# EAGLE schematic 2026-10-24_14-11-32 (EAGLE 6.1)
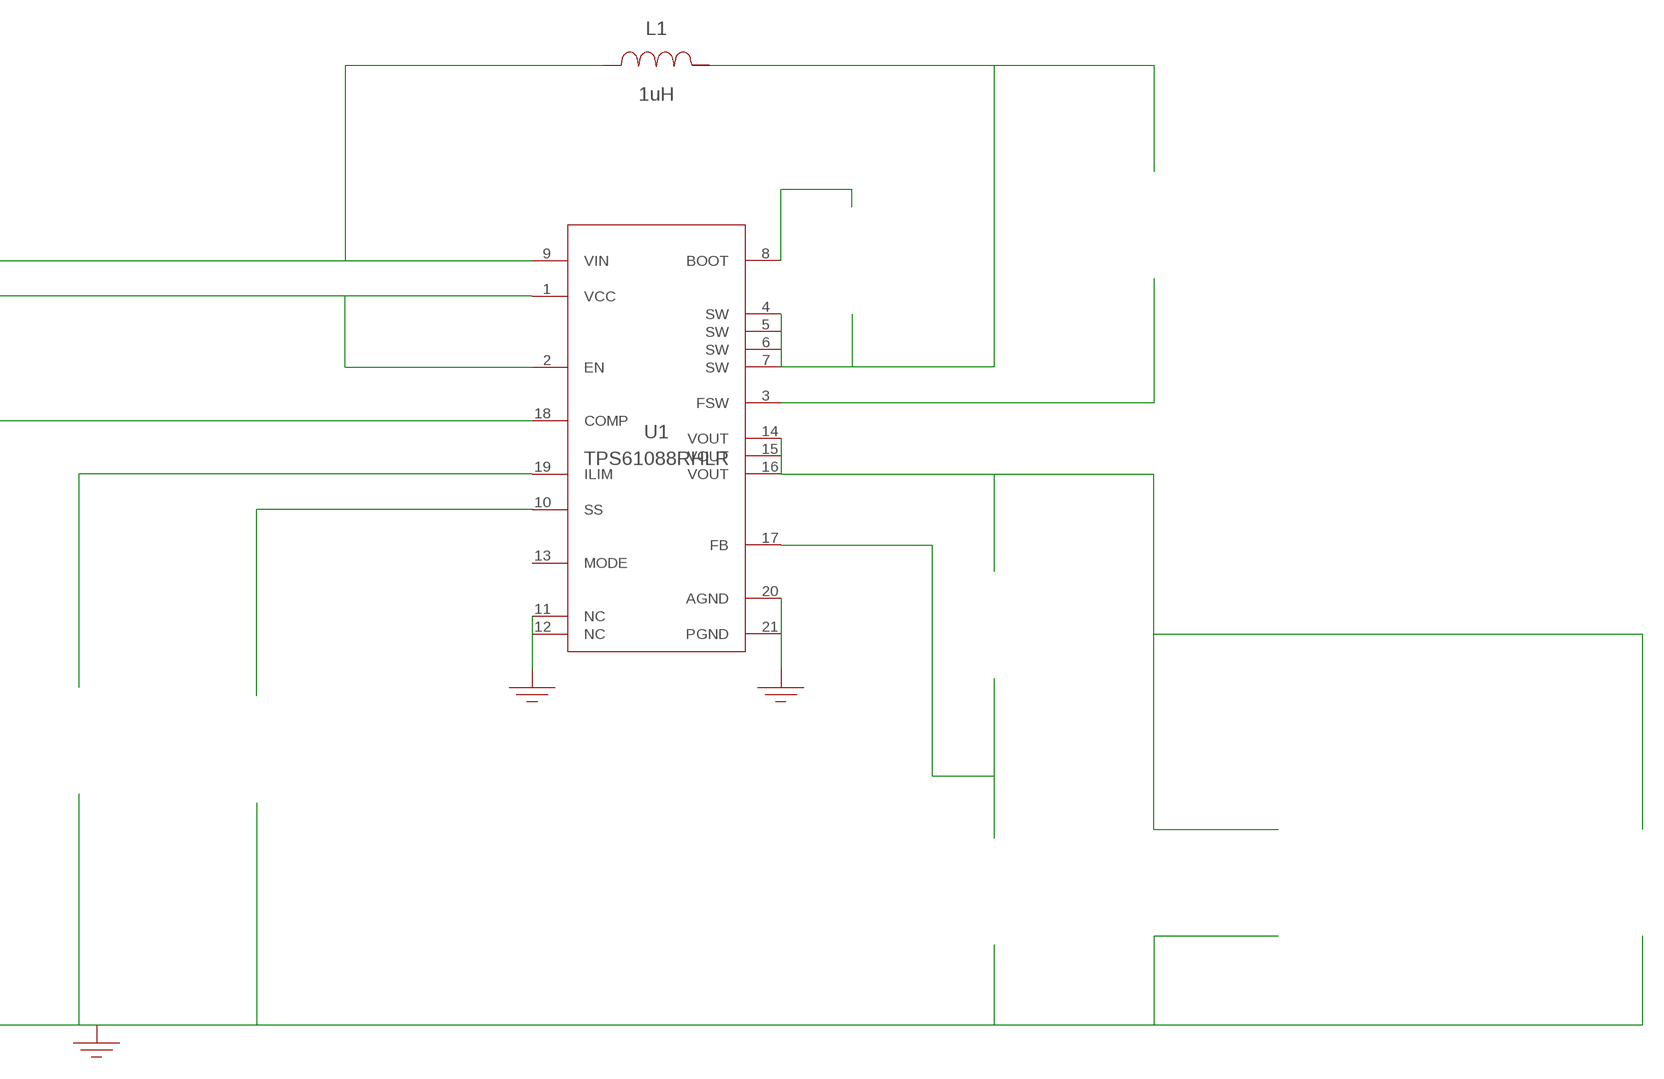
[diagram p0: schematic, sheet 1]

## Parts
CBST  100nF  08053C104KAT2A08053C104KAT2A  [0805]  (not placed on a sheet)
CCOMP  750pF  GRM1555C1E751JA01DGRM1555C1E751JA01D  [0402]  (not placed on a sheet)
CCOMP2  39pF  GRM1555C1E390JA01DGRM1555C1E390JA01D  [0402]  (not placed on a sheet)
CIN  10uF  MSASE21GAB5106KTNA01MSASE21GAB5106KTNA01  [0805]  (not placed on a sheet)
CIN2  100nF  GRM155R71A104KA01DGRM155R71A104KA01D  [0402]  (not placed on a sheet)
CIN_2  10uF  MSASE21GAB5106KTNA01MSASE21GAB5106KTNA01  [0805]  (not placed on a sheet)
CIN_3  10uF  MSASE21GAB5106KTNA01MSASE21GAB5106KTNA01  [0805]  (not placed on a sheet)
COUT  47uF  GRM32ER61C476KE15LGRM32ER61C476KE15L  [1210_280]  (not placed on a sheet)
COUT_2  47uF  GRM32ER61C476KE15LGRM32ER61C476KE15L  [1210_280]  (not placed on a sheet)
CSS  8.2nF  GRM155R71C822KA01DGRM155R71C822KA01D  [0402]  (not placed on a sheet)
CVCC  1uF  EMK107B7105KA-TEMK107B7105KA-T  [0603]  (not placed on a sheet)
CVCC_2  1uF  EMK107B7105KA-TEMK107B7105KA-T  [0603]  (not placed on a sheet)
GND1  WB_GND  WB_GNDWB_GND  [WB_GND]
GND2  WB_GND  WB_GNDWB_GND  [WB_GND]
GND3  WB_GND  WB_GNDWB_GND  [WB_GND]
IOUT  WB_CURRENT_LOAD  WB_CURRENT_LOADWB_CURRENT_LOAD  [WB_CURRENT_LOAD]  (not placed on a sheet)
L1  1uH  VLP8040T-1R0NVLP8040T-1R0N  [VLP8040]
RCOMP  26.7k  CRCW040226K7FKEDCRCW040226K7FKED  [0402]  (not placed on a sheet)
RFBB  69.8k  CRCW040269K8FKEDCRCW040269K8FKED  [0402]  (not placed on a sheet)
RFBT  220k  RC0603FR-07220KLRC0603FR-07220KL  [0603]  (not placed on a sheet)
RLIM  154k  CRCW0402154KFKEDCRCW0402154KFKED  [0402]  (not placed on a sheet)
RT  267k  CRCW0402267KFKEDCRCW0402267KFKED  [0402]  (not placed on a sheet)
U1  TPS61088RHLR  TPS61088RHLRTPS61088RHLR  [RHL0020A]
VIN  WB_BATTERY  WB_BATTERYWB_BATTERY  [WB_BATTERY]  (not placed on a sheet)
Unconnected: CBST.1 CBST.2 CCOMP2.1 CCOMP2.2 CCOMP.1 CCOMP.2 CIN2.1 CIN2.2 CIN.1 CIN.2 CIN_2.1 CIN_2.2 CIN_3.1 CIN_3.2 COUT.1 COUT.2 COUT_2.1 COUT_2.2 CSS.1 CSS.2 CVCC.1 CVCC.2 CVCC_2.1 CVCC_2.2 GND1.1 GND2.1 GND3.1 IOUT.1(+) IOUT.2(-) L1.1 L1.2 RCOMP.1 RCOMP.2 RFBB.1 RFBB.2 RFBT.1 RFBT.2 RLIM.1 RLIM.2 RT.1 RT.2 U1.2(EN) U1.3(FSW) U1.10(SS) U1.11(NC) U1.12(NC) U1.13(MODE) U1.17(FB) U1.18(COMP) U1.19(ILIM) VIN.1(+) VIN.2(-)

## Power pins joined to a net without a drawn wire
AGND: U1.20(AGND)
BOOT: U1.8(BOOT)
PGND: U1.21(PGND)
SW: U1.4(SW) U1.5(SW) U1.6(SW) U1.7(SW)
VCC: U1.1(VCC)
VIN: U1.9(VIN)
VOUT: U1.14(VOUT) U1.15(VOUT) U1.16(VOUT)

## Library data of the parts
CBST = AcceleratedDesigns_Lib:08053C104KAT2A; Manufacturer_Part_Number: 08053C104KAT2A; Vendor: AVX
CCOMP = AcceleratedDesigns_Lib:GRM1555C1E751JA01D; Manufacturer_Part_Number: GRM1555C1E751JA01D; Vendor: MuRata
CCOMP2 = AcceleratedDesigns_Lib:GRM1555C1E390JA01D; Manufacturer_Part_Number: GRM1555C1E390JA01D; Vendor: MuRata
CIN CIN_2 CIN_3 = AcceleratedDesigns_Lib:MSASE21GAB5106KTNA01; Manufacturer_Part_Number: MSASE21GAB5106KTNA01; Vendor: Taiyo Yuden
CIN2 = AcceleratedDesigns_Lib:GRM155R71A104KA01D; Manufacturer_Part_Number: GRM155R71A104KA01D; Vendor: MuRata
COUT COUT_2 = AcceleratedDesigns_Lib:GRM32ER61C476KE15L; Manufacturer_Part_Number: GRM32ER61C476KE15L; Vendor: MuRata
CSS = AcceleratedDesigns_Lib:GRM155R71C822KA01D; Manufacturer_Part_Number: GRM155R71C822KA01D; Vendor: MuRata
CVCC CVCC_2 = AcceleratedDesigns_Lib:EMK107B7105KA-T; Manufacturer_Part_Number: EMK107B7105KA-T; Vendor: Taiyo Yuden
GND1-GND3 = AcceleratedDesigns_Lib:WB_GND; Manufacturer_Part_Number: WB_GND
IOUT = AcceleratedDesigns_Lib:WB_CURRENT_LOAD; Manufacturer_Part_Number: WB_CURRENT_LOAD
L1 = AcceleratedDesigns_Lib:VLP8040T-1R0N; Manufacturer_Part_Number: VLP8040T-1R0N; Vendor: TDK
RCOMP = AcceleratedDesigns_Lib:CRCW040226K7FKED; Manufacturer_Part_Number: CRCW040226K7FKED; Vendor: Vishay-Dale
RFBB = AcceleratedDesigns_Lib:CRCW040269K8FKED; Manufacturer_Part_Number: CRCW040269K8FKED; Vendor: Vishay-Dale
RFBT = AcceleratedDesigns_Lib:RC0603FR-07220KL; Manufacturer_Part_Number: RC0603FR-07220KL; Vendor: Yageo America
RLIM = AcceleratedDesigns_Lib:CRCW0402154KFKED; Manufacturer_Part_Number: CRCW0402154KFKED; Vendor: Vishay-Dale
RT = AcceleratedDesigns_Lib:CRCW0402267KFKED; Manufacturer_Part_Number: CRCW0402267KFKED; Vendor: Vishay-Dale
U1 = AcceleratedDesigns_Lib:TPS61088RHLR; Manufacturer_Part_Number: TPS61088RHLR
VIN = AcceleratedDesigns_Lib:WB_BATTERY; Manufacturer_Part_Number: WB_BATTERY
